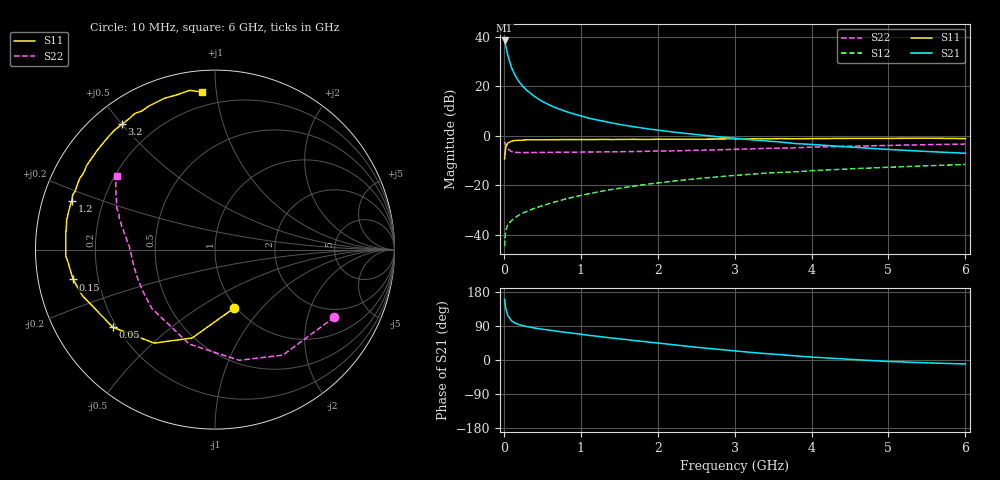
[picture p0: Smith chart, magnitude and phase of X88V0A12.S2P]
! SIEMENS Small Signal Semiconductors
! BFP136W
! Si NPN RF Bipolar Junction Transistor in SOT343
! VCE = 8 V  IC = 120 mA
! Common Emitter S-Parameters:  September  1994
# GHz  S  MA  R  50
!  f  S11  S21  S12  S22
! GHz  MAG  ANG  MAG  ANG  MAG  ANG  MAG  ANG
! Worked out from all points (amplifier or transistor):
!   40 points, 10 MHz to 6 GHz, reference 50 ohm
!   highest |S21| = 38.6 dB at 10 MHz (marker M1)
!   |S21| within 3 dB of that: start of sweep to 30.94 MHz
!   unconditionally stable (mu >= 1): 606.7 MHz to 3.323 GHz; 3.756 GHz to 3.844 GHz
!   at 200 MHz: K = 0.67, MSG = 26.9 dB, |S12| = -31.9 dB
!   at 1.5 GHz: K = 1.11, MAG = 10.9 dB, |S12| = -21.2 dB
!   at 6 GHz: K = 0.97, MSG = 2.3 dB, |S12| = -11.5 dB
!   S11 on the Smith chart (normalised r, x): 10 MHz: 0.97, -0.72; 50 MHz: 0.18, -0.33; 150 MHz: 0.11, -0.10; 1.2 GHz: 0.09, +0.16; 3.2 GHz: 0.09, +0.50; 6 GHz: 0.12, +0.91
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0.01  0.3436 -72.4  84.86 160.0  0.0059 68.9  0.7643 -29.5
0.02  0.5085 -104.5  72.48 143.5  0.0103 56.0  0.6989 -57.3
0.03  0.6213 -123.0  61.05 131.8  0.013 49.9  0.6312 -77.7
0.05  0.7151 -142.8  43.39 117.7  0.0159 40.1  0.5456 -105.2
0.1  0.7828 -161.0  23.94 103.4  0.0195 37.7  0.4811 -136.9
0.15  0.8074 -168.1  16.29 97.1  0.0224 39.6  0.4643 -150.0
0.2  0.8148 -172.2  12.26 93.2  0.0253 41.2  0.4603 -157.1
0.25  0.8223 -175.3  9.89 90.4  0.0277 43.1  0.46 -161.7
0.3  0.8315 -177.4  8.275 88.3  0.0298 44.6  0.4595 -164.8
0.4  0.8313 178.5  6.237 84.4  0.0345 47.9  0.4617 -169.0
0.5  0.8332 175.7  4.979 81.2  0.0386 50.2  0.4632 -171.9
0.6  0.8361 173.6  4.153 78.6  0.0434 51.9  0.4644 -173.7
0.7  0.8381 170.9  3.579 75.5  0.0479 53.6  0.4661 -175.1
0.9  0.8419 167.1  2.804 70.5  0.0577 55.2  0.4684 -177.7
1.1  0.8433 162.7  2.294 65.1  0.0675 56.5  0.472 -179.4
1.2  0.8425 161.3  2.117 63.0  0.0723 56.7  0.4744 179.9
1.6  0.8496 153.8  1.608 53.8  0.092 56.0  0.4818 176.8
2.2  0.8552 143.5  1.197 40.4  0.1215 52.7  0.498 172.6
3.2  0.8698 126.5  0.84 20.3  0.1672 44.4  0.5441 164.2
4.5  0.8889 108.5  0.595 1.8  0.2154 33.6  0.6169 153.0
5.5  0.8986 99.1  0.484 -7.5  0.2485 25.6  0.6647 146.3
6  0.8813 94.8  0.446 -10.5  0.265 21.4  0.6821 143.3
